{attribute 'Tc2GvlVarNames'}
(* Generated automatically by TwinCAT - (read only) *)
VAR_CONFIG
	.WebTransport.PlcToNc AT %QB0 : PLCTONC_AXIS_REF;	(*  ~ {LinkedWith:TINC^NC-Task 1 SAF^Axes^WebTransport^Inputs^WebTransport_FromPlc} *)
	.WebTransport.NcToPlc AT %IB0 : NCTOPLC_AXIS_REF;	(*  ~ {LinkedWith:TINC^NC-Task 1 SAF^Axes^WebTransport^Outputs^WebTransport_ToPlc} *)
	.VirtualWeb.PlcToNc AT %QB128 : PLCTONC_AXIS_REF;	(*  ~ {LinkedWith:TINC^NC-Task 1 SAF^Axes^VirtualWeb^Inputs^VirtualWeb_FromPlc} *)
	.VirtualWeb.NcToPlc AT %IB128 : NCTOPLC_AXIS_REF;	(*  ~ {LinkedWith:TINC^NC-Task 1 SAF^Axes^VirtualWeb^Outputs^VirtualWeb_ToPlc} *)
	.RotaryKnife.PlcToNc AT %QB256 : PLCTONC_AXIS_REF;	(*  ~ {LinkedWith:TINC^NC-Task 1 SAF^Axes^RotaryKnife^Inputs^RotaryKnife_FromPlc} *)
	.RotaryKnife.NcToPlc AT %IB256 : NCTOPLC_AXIS_REF;	(*  ~ {LinkedWith:TINC^NC-Task 1 SAF^Axes^RotaryKnife^Outputs^RotaryKnife_ToPlc} *)
END_VAR
